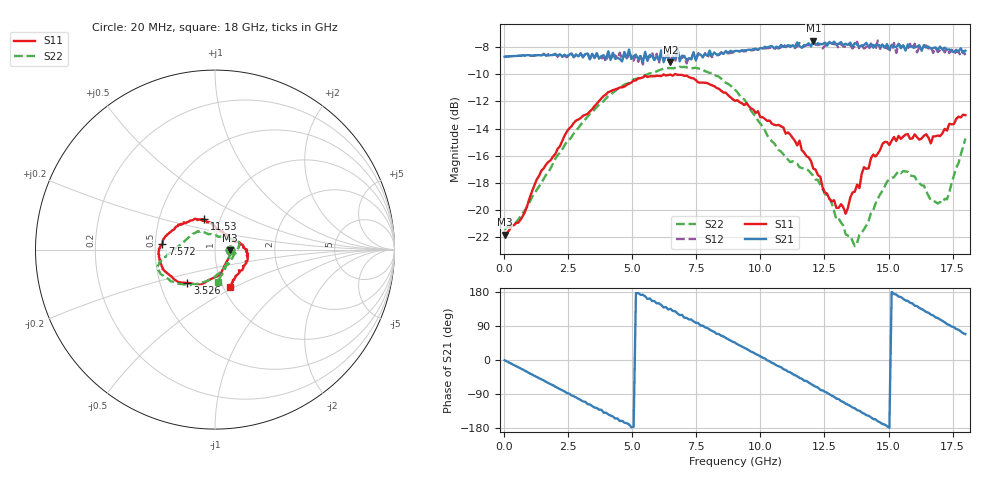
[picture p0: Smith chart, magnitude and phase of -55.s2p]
!Agilent Technologies,N5230A,US43500223,A.07.50.48
!Agilent N5230A: A.07.50.48
!Date: Wednesday, January 13, 2016 16:13:16
!Correction: S11(Full 2 Port(1,2))
!S21(Full 2 Port(1,2))
!S12(Full 2 Port(1,2))
!S22(Full 2 Port(1,2))
!S2P File: Measurements: S11, S21, S12, S22:
# Hz S  dB  R 50
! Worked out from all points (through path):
!   201 points, 20 MHz to 18 GHz, reference 50 ohm
!   highest |S21| = -7.55 dB at 12.07 GHz (marker M1); lowest = -9.1 dB at 6.493 GHz (marker M2)
!   group delay of S21, straight-line fit = 100 ps
!   lowest |S11| = -21.8 dB at 20 MHz (marker M3), VSWR 1.18, Z = 58.8 - j0.465 ohm
!   |S11| at or under -10 dB: start of sweep to 6.662 GHz; 6.694 GHz to end of sweep
!   |S22| runs from -22.6 to -9.5 dB; largest |S21 - S12| = 0.053
!   S11 on the Smith chart (normalised r, x): 20 MHz: 1.18, -0.01; 3.526 GHz: 0.69, -0.27; 7.572 GHz: 0.55, +0.04; 11.53 GHz: 0.84, +0.29; 18 GHz: 1.07, -0.47
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2e7  -21.80 -2.8  -8.71 -0.7  -8.72 -0.8  -21.43 -1.9
9.19e8  -19.57 -59.9  -8.60 -31.9  -8.61 -32.3  -19.69 -52.9
1.818e9  -16.32 -89.7  -8.60 -64.1  -8.58 -65.3  -16.92 -86.7
3.0766e9  -13.06 -118.5  -8.77 -109.5  -8.70 -110.1  -13.50 -116.4
3.5261e9  -12.35 -129.6  -8.78 -125.5  -8.82 -127.1  -12.62 -123.7
4.8746e9  -10.70 -151.2  -8.18 -170.0  -8.50 -170.6  -10.64 -142.2
6.0433e9  -10.13 -166.7  -8.96 149.6  -9.22 145.9  -9.72 -154.3
6.4928e9  -10.03 -173.1  -9.13 135.0  -9.08 131.1  -9.56 -157.6
6.7625e9  -10.05 -176.4  -8.08 123.1  -8.36 121.7  -9.53 -159.8
6.8524e9  -10.05 -177.5  -9.06 118.4  -8.79 115.0  -9.46 -160.2
7.5716e9  -10.60 173.8  -8.52 97.8  -8.47 96.1  -9.58 -163.8
9.01e9  -11.96 152.8  -8.30 45.8  -8.35 42.9  -11.15 -171.8
1.03585e10  -13.41 131.1  -7.97 -3.4  -8.07 -6.9  -14.71 168.4
1.15272e10  -14.88 109.6  -7.95 -47.2  -7.70 -50.3  -16.84 139.8
1.20666e10  -16.94 95.6  -7.55 -66.7  -7.77 -69.8  -17.46 131.0
1.33252e10  -20.26 39.7  -7.76 -114.8  -7.97 -117.7  -21.76 97.1
1.36848e10  -18.64 24.9  -7.71 -127.5  -7.94 -129.7  -22.64 76.5
1.45838e10  -15.83 4.9  -7.85 -162.0  -7.52 -165.1  -19.15 32.3
1.50333e10  -15.21 -2.9  -8.18 -178.9  -8.20 176.2  -17.74 22.5
1.60222e10  -14.42 -23.1  -8.04 143.4  -7.75 141.0  -17.53 5.3
1.7101e10  -14.35 -54.4  -8.19 103.5  -8.02 96.9  -19.46 -40.7
1.8e10  -13.01 -68.5  -8.27 68.3  -8.60 62.4  -14.73 -84.7
